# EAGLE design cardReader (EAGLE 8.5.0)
DELETE: MF
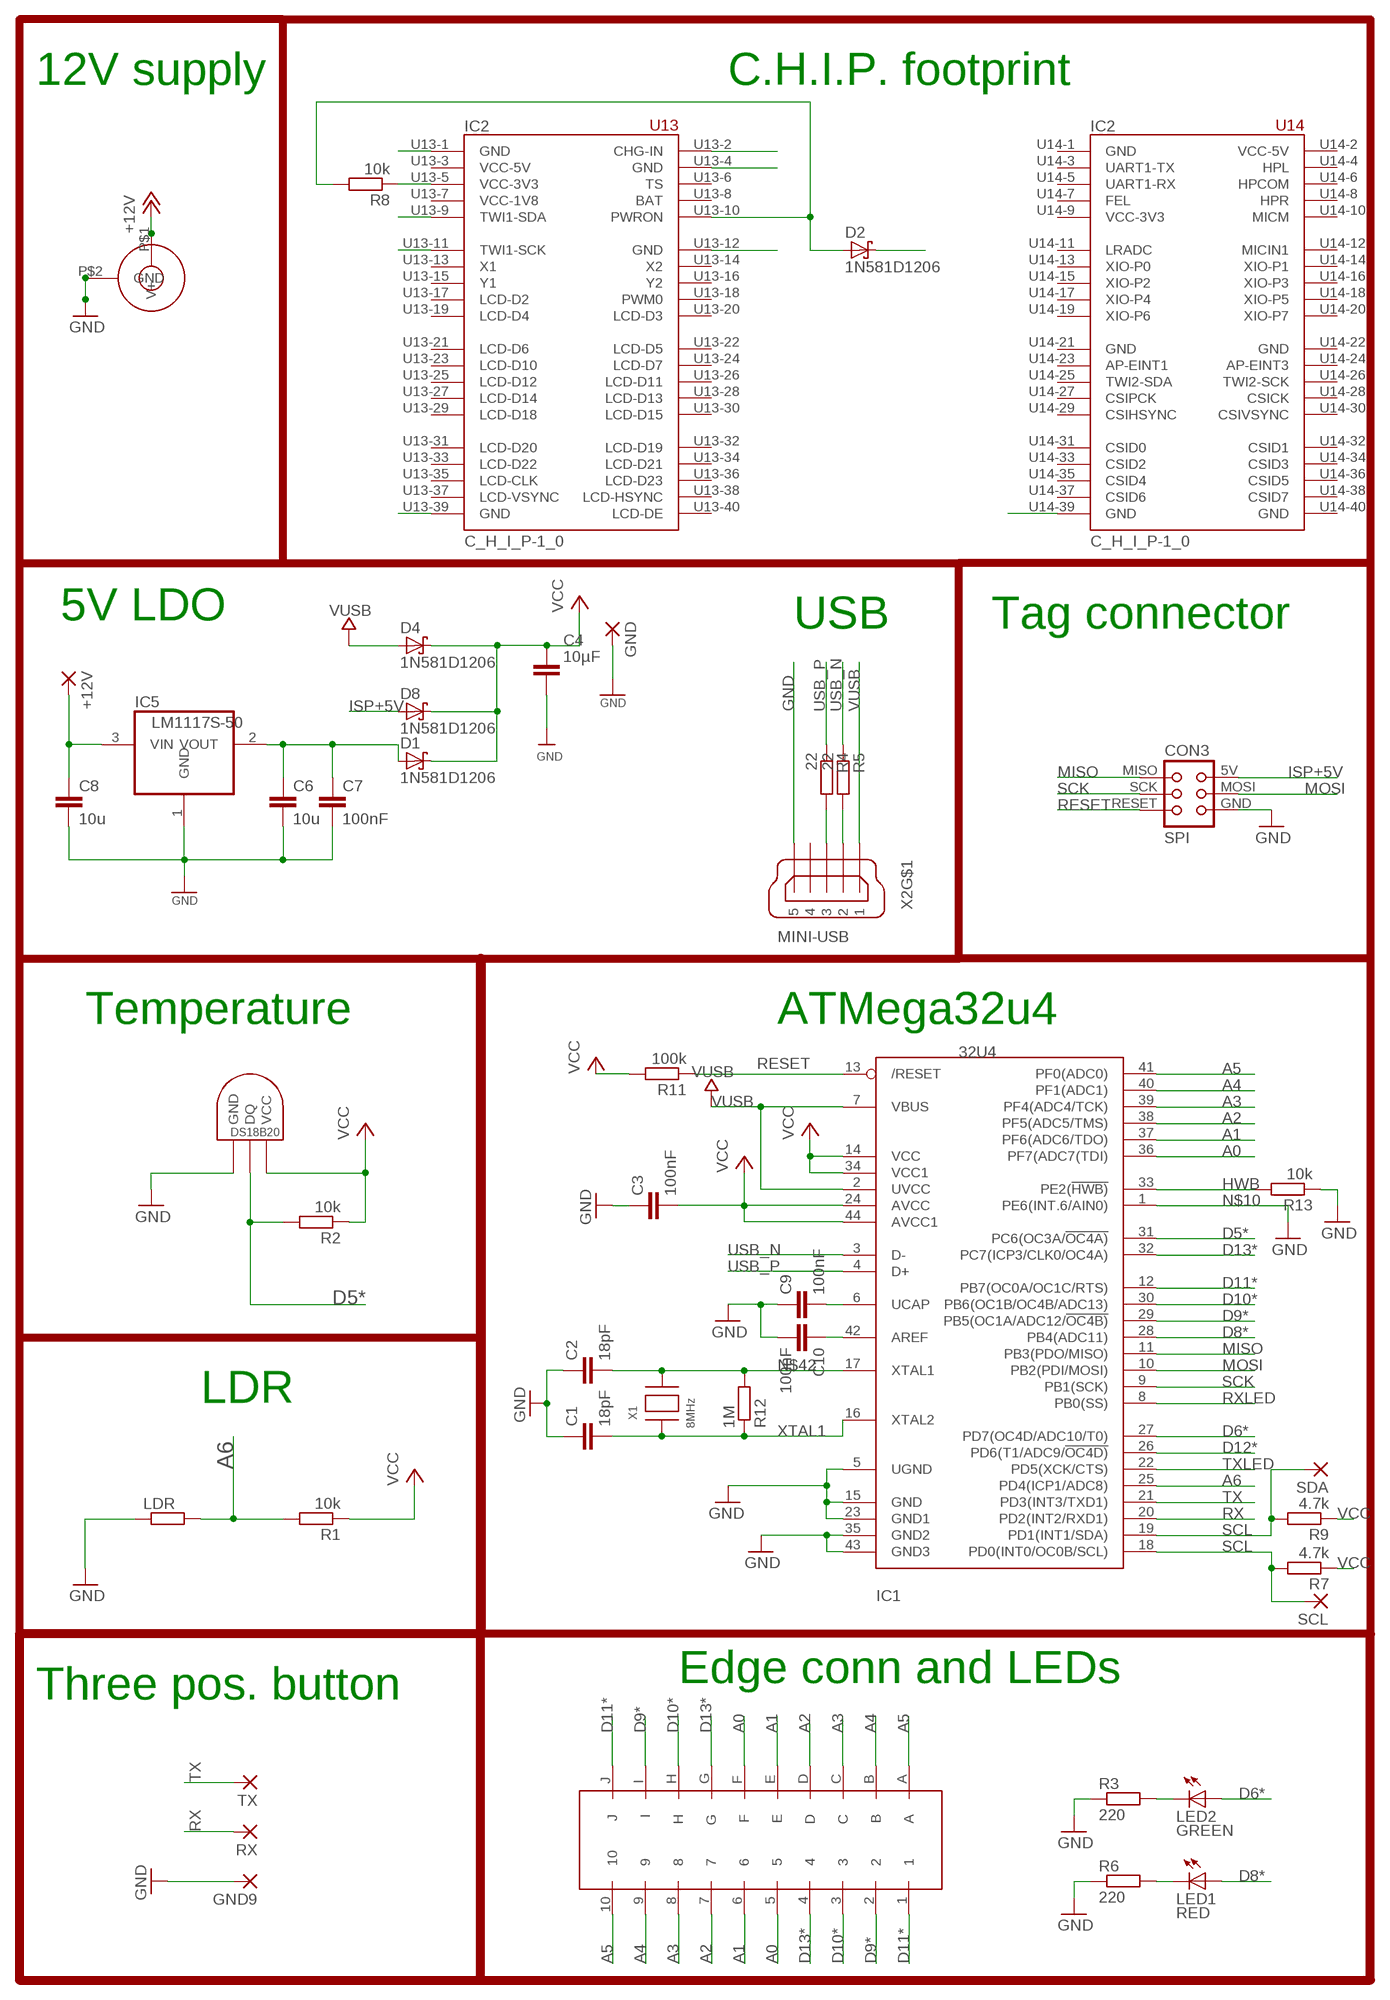
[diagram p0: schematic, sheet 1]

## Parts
+12V  SMD5  [SMD2,54-5,08]
C1  18pF  C-EUC0805K  [C0805K]
C2  18pF  C-EUC0805K  [C0805K]
C3  100nF  C-EUC0805K  [C0805K]
C4  10µF  CAPACITOR_NPOL-1206  [C1206]
C6  10u  C-EUC0805K  [C0805K]
C7  100nF  C-EUC0805K  [C0805K]
C8  10u  C-EUC0805K  [C0805K]
C9  100nF  C-EUC0805K  [C0805K]
C10  100nF  C-EUC0805K  [C0805K]
CON2  JACK_DC_BARREL  [DC_BARREL]
CON3  SPI  TINYISPT  [TC2030-MCP-NL]
D1  1N581D1206  [LED-1206]
D2  1N581D1206  [LED-1206]
D4  1N581D1206  [LED-1206]
D8  1N581D1206  [LED-1206]
GND  SMD5  [SMD2,54-5,08]
GND9  SMD5  [SMD2,54-5,08]
IC1  32U4  ATMEGA32U4-AU  [TQFP44]
IC2  C_H_I_P-1_0  [C_H_I_P-1_0]
IC5  LM1117S-50  REG1117  [SOT223]
LDR  R-EU_0207/2V  [0207/2V]
LED1  RED  LED5MM  [LED5MM]
LED2  GREEN  LED5MM  [LED5MM]
R1  10k  R-EU_R0805  [R0805]
R2  10k  R-EU_R0805  [R0805]
R3  220  R-EU_0204/7  [0204/7]
R4  22  R-EU_R0805  [R0805]
R5  22  R-EU_R0805  [R0805]
R6  220  R-EU_0204/7  [0204/7]
R7  4.7k  R-EU_R0805  [R0805]
R8  10k  R-EU_R0805  [R0805]
R9  4.7k  R-EU_R0805  [R0805]
R11  100k  R-EU_R0805  [R0805]
R12  1M  R-EU_R0805  [R0805]
R13  10k  R-EU_R0805  [R0805]
RX  SMD5  [SMD2,54-5,08]
SCL  SMD5  [SMD2,54-5,08]
SDA  SMD5  [SMD2,54-5,08]
TX  SMD5  [SMD2,54-5,08]
U$1  DS1820TO92  [DS1820]
U$3  CONN2X10PRINT  [CONN2X10PRINT]
X1  8MHz  XTALNX6035  [NX6035]
X2  MINI-USB  MINI-USB-SCHIELD-32005-201  [32005-201]

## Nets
+12V: +12V.1(P) C8.1 CON2.P$1(V+) IC5.3(VIN)
A0: IC1.36(PF7(ADC7(TDI)) U$3.5 U$3.F
A1: IC1.37(PF6(ADC6/TDO)) U$3.6 U$3.E
A2: IC1.38(PF5(ADC5/TMS)) U$3.7 U$3.D
A3: IC1.39(PF4(ADC4/TCK)) U$3.8 U$3.C
A4: IC1.40(PF1(ADC1)) U$3.9 U$3.B
A5: IC1.41(PF0(ADC0)) U$3.10 U$3.A
A6: IC1.25(PD4(ICP1/ADC8)) LDR.2 R1.2
AREF: C10.1 IC1.42(AREF)
D5*: IC1.31(PC6(OC3A/!OC4A)) R2.2 U$1.DQ
D6*: IC1.27(PD7(OC4D/ADC10/T0)) LED2.A
D8*: IC1.28(PB4(ADC11)) LED1.A
D9*: IC1.29(PB5(OC1A/ADC12/!OC4B)) U$3.2 U$3.I
D10*: IC1.30(PB6(OC1B/OC4B/ADC13)) U$3.3 U$3.H
D11*: IC1.12(PB7(OC0A/OC1C/RTS)) U$3.1 U$3.J
D12*: IC1.26(PD6(T1/ADC9/!OC4D))
D13*: IC1.32(PC7(ICP3/CLK0/OC4A)) U$3.4 U$3.G
GND [power]: C1.1 C2.1 C3.1 C4.2 C6.2 C7.2 C8.2 C9.1 C10.2 CON2.P$2(GND) CON3.GND GND9.1(P) GND.1(P) IC1.5(UGND) IC1.15(GND) IC1.23(GND1) IC1.35(GND2) IC1.43(GND3) IC2.U13-12(GND) IC2.U13-39(GND) IC5.1(GND) LDR.1 R3.1 R6.1 R13.1 U$1.GND X2.5
HWB: IC1.33(PE2(!HWB)) R13.2
ISP+5V: CON3.5V(VCC) D8.A
MISO: CON3.MISO IC1.11(PB3(PDO/MISO))
MOSI: CON3.MOSI IC1.10(PB2(PDI/MOSI))
N$1: C9.2 IC1.6(UCAP)
N$2: IC2.U13-2(CHG-IN)
N$3: LED2.K(C) R3.2
N$4: LED1.K(C) R6.2
N$5: IC2.U13-4(GND)
N$6: IC2.U13-1(GND)
N$7: IC2.U13-9(TWI1-SDA)
N$8: IC2.U13-11(TWI1-SCK)
N$9: C6.1 C7.1 D1.A IC5.2(VOUT)
N$10: D2.C IC1.1(PE6(INT.6/AIN0)) ; supply symbol labelled GND
N$11: IC2.U14-39(GND)
N$42: C2.2 IC1.17(XTAL1) R12.2 X1.P$2
PWRON: D2.A IC2.U13-10(PWRON) R8.2
RESET: CON3.RESET IC1.13(/RESET) R11.1
RX: IC1.20(PD2(INT2/RXD1)) RX.1(P)
RXLED: IC1.8(PB0(SS))
SCK: CON3.SCK IC1.9(PB1(SCK))
SCL: IC1.18(PD0(INT0/OC0B/SCL)) R7.2 SCL.1(P)
SDA: IC1.19(PD1(INT1/SDA)) R9.2 SDA.1(P)
TX: IC1.21(PD3(INT3/TXD1)) TX.1(P)
TXLED: IC1.22(PD5(XCK/CTS))
USB_N: IC1.3(D-) R5.1
USB_P: IC1.4(D+) R4.1
USBC_N: R5.2 X2.2
USBC_P: R4.2 X2.3
VCC: C3.2 C4.1 D1.C D4.C D8.C IC1.14(VCC) IC1.24(AVCC) IC1.34(VCC1) IC1.44(AVCC1) R1.1 R2.1 R7.1 R9.1 R11.2 U$1.VDD(VCC)
VCC-3V3@1: IC2.U13-5(VCC-3V3) R8.1
VUSB: D4.A IC1.2(UVCC) IC1.7(VBUS) X2.1
XTAL1: C1.2 IC1.16(XTAL2) R12.1 X1.P$1
Unconnected: IC2.U13-3(VCC-5V) IC2.U13-6(TS) IC2.U13-7(VCC-1V8) IC2.U13-13(X1) IC2.U13-14(X2) IC2.U13-15(Y1) IC2.U13-16(Y2) IC2.U13-17(LCD-D2) IC2.U13-18(PWM0) IC2.U13-19(LCD-D4) IC2.U13-20(LCD-D3) IC2.U13-21(LCD-D6) IC2.U13-22(LCD-D5) IC2.U13-23(LCD-D10) IC2.U13-24(LCD-D7) IC2.U13-25(LCD-D12) IC2.U13-26(LCD-D11) IC2.U13-27(LCD-D14) IC2.U13-28(LCD-D13) IC2.U13-29(LCD-D18) IC2.U13-30(LCD-D15) IC2.U13-31(LCD-D20) IC2.U13-32(LCD-D19) IC2.U13-33(LCD-D22) IC2.U13-34(LCD-D21) IC2.U13-35(LCD-CLK) IC2.U13-36(LCD-D23) IC2.U13-37(LCD-VSYNC) IC2.U13-38(LCD-HSYNC) IC2.U13-40(LCD-DE) IC2.U14-2(VCC-5V) IC2.U14-3(UART1-TX) IC2.U14-4(HPL) IC2.U14-5(UART1-RX) IC2.U14-6(HPCOM) IC2.U14-7(FEL) IC2.U14-8(HPR) IC2.U14-9(VCC-3V3) IC2.U14-10(MICM) IC2.U14-11(LRADC) IC2.U14-12(MICIN1) IC2.U14-13(XIO-P0) IC2.U14-14(XIO-P1) IC2.U14-15(XIO-P2) IC2.U14-16(XIO-P3) IC2.U14-17(XIO-P4) IC2.U14-18(XIO-P5) IC2.U14-19(XIO-P6) IC2.U14-20(XIO-P7) IC2.U14-23(AP-EINT1) IC2.U14-24(AP-EINT3) IC2.U14-25(TWI2-SDA) IC2.U14-26(TWI2-SCK) IC2.U14-27(CSIPCK) IC2.U14-28(CSICK) IC2.U14-29(CSIHSYNC) IC2.U14-30(CSIVSYNC) IC2.U14-31(CSID0) IC2.U14-32(CSID1) IC2.U14-33(CSID2) IC2.U14-34(CSID3) IC2.U14-35(CSID4) IC2.U14-36(CSID5) IC2.U14-37(CSID6) IC2.U14-38(CSID7) X2.4 X2.M1(S:S1) X2.M2(S:S2) X2.M3(S:S3) X2.M4(S:S4)

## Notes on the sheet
- 12V supply | C.H.I.P. footprint
- 5V LDO | USB | Tag connector
- Temperature | ATMega32u4
- LDR
- Edge conn and LEDs
- Three pos. button

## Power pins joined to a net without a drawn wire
BAT: IC2.U13-8(BAT)
GND: IC2.U14-1(GND) IC2.U14-21(GND) IC2.U14-22(GND) IC2.U14-40(GND)

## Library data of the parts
+12V GND GND9 RX SCL SDA TX = wirepad:SMD5: SMD PAD
C1 C2 = rcl:C-EU: CAPACITOR, European symbol; ELECROW: C1797; LCSC: C1797; MPN: 77-VJ1206A180JXXPBC
C3 C7 C9 C10 = rcl:C-EU: CAPACITOR, European symbol; ELECROW: C49678; LCSC: C49678; MPN: 80-C1206C104K5R
C4 = dp_devices:CAPACITOR_NPOL: Non-Polarized capacitor in various packages
C6 C8 = rcl:C-EU: CAPACITOR, European symbol; ELECROW: C15850; LCSC: C15850; MPN: 77-VJ1206V106ZXQTBC
CON2 = lpatiny:JACK_DC_BARREL
CON3 = lpatiny:TINYISP: CONNECTOR
D1 D2 D4 D8 = lpatiny:1N581*: 1.0A SCHOTTKY BARRIER RECTIFIER
IC1 = adafruit:ATMEGA32U4: http://www.ladyada.net/library/eagle; LCSC: C44854; MPN: 556-ATMEGA32U4RC-AU
IC2 = SENG:C_H_I_P-1_0: C.H.I.P. 1.0 Linux computer module with on chip power management unit
IC5 = burr-brown:REG1117: 800mA and 1A Low Dropout (LDO) Positive Regulator 1.8V, 2.5V, 2.85V, 3.3V, 5V, and Adj; LCSC: C126027; MPN: REG1117; OC_FARNELL: 1097566; OC_NEWARK: 14P6981
LDR R3 R6 = rcl:R-EU_: RESISTOR, European symbol
LED1 LED2 = SparkFun:LED: LEDs
R1 R2 R7-R9 R11 = rcl:R-EU_: RESISTOR, European symbol; ELECROW: C17407; LCSC: C17407; MPN: RC1206FR-07100KL
R4 R5 = rcl:R-EU_: RESISTOR, European symbol; ELECROW: C17561; LCSC: C17561
R12 = rcl:R-EU_: RESISTOR, European symbol; ELECROW: C17514; LCSC: C17514
R13 = rcl:R-EU_: RESISTOR, European symbol; ELECROW: C17414; LCSC: C17414
U$1 = Ava:DS1820: DS18B20 Programmable Resolution 1-Wire Digital Thermometer Description The DS18B20 digital thermometer provides 9-bit to 12-bit Celsius temperature measurements and has an alarm function with nonvolatile user-programmable upper and lower trigger points. The DS18B20 communicates over a 1-Wire® bus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
U$3 = edgeConn2x10:CONN2X10PRINT: Footprint for 10/20 edge connector.
X1 = lpatiny:XTAL: Low cost SMT crystals, no capacitors included; LCSC: C122522; MPN: 729-F60800010
X2 = con-cypressindustries:MINI-USB-SCHIELD-: MINI USB-B Conector Source: www.cypressindustries.com; LCSC: C46391; MPN: 649-10033526-N3212LF

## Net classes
0 default: width 0.254 mm, clearance 0.25 mm
1 power: width 0.254 mm, drill 0.305 mm, clearance 0.25 mm
2 VIN: width 0.254 mm, clearance 0.25 mm
3 fine: width 0.254 mm, clearance 0.25 mm
4 aref: width 0.254 mm, clearance 0.25 mm

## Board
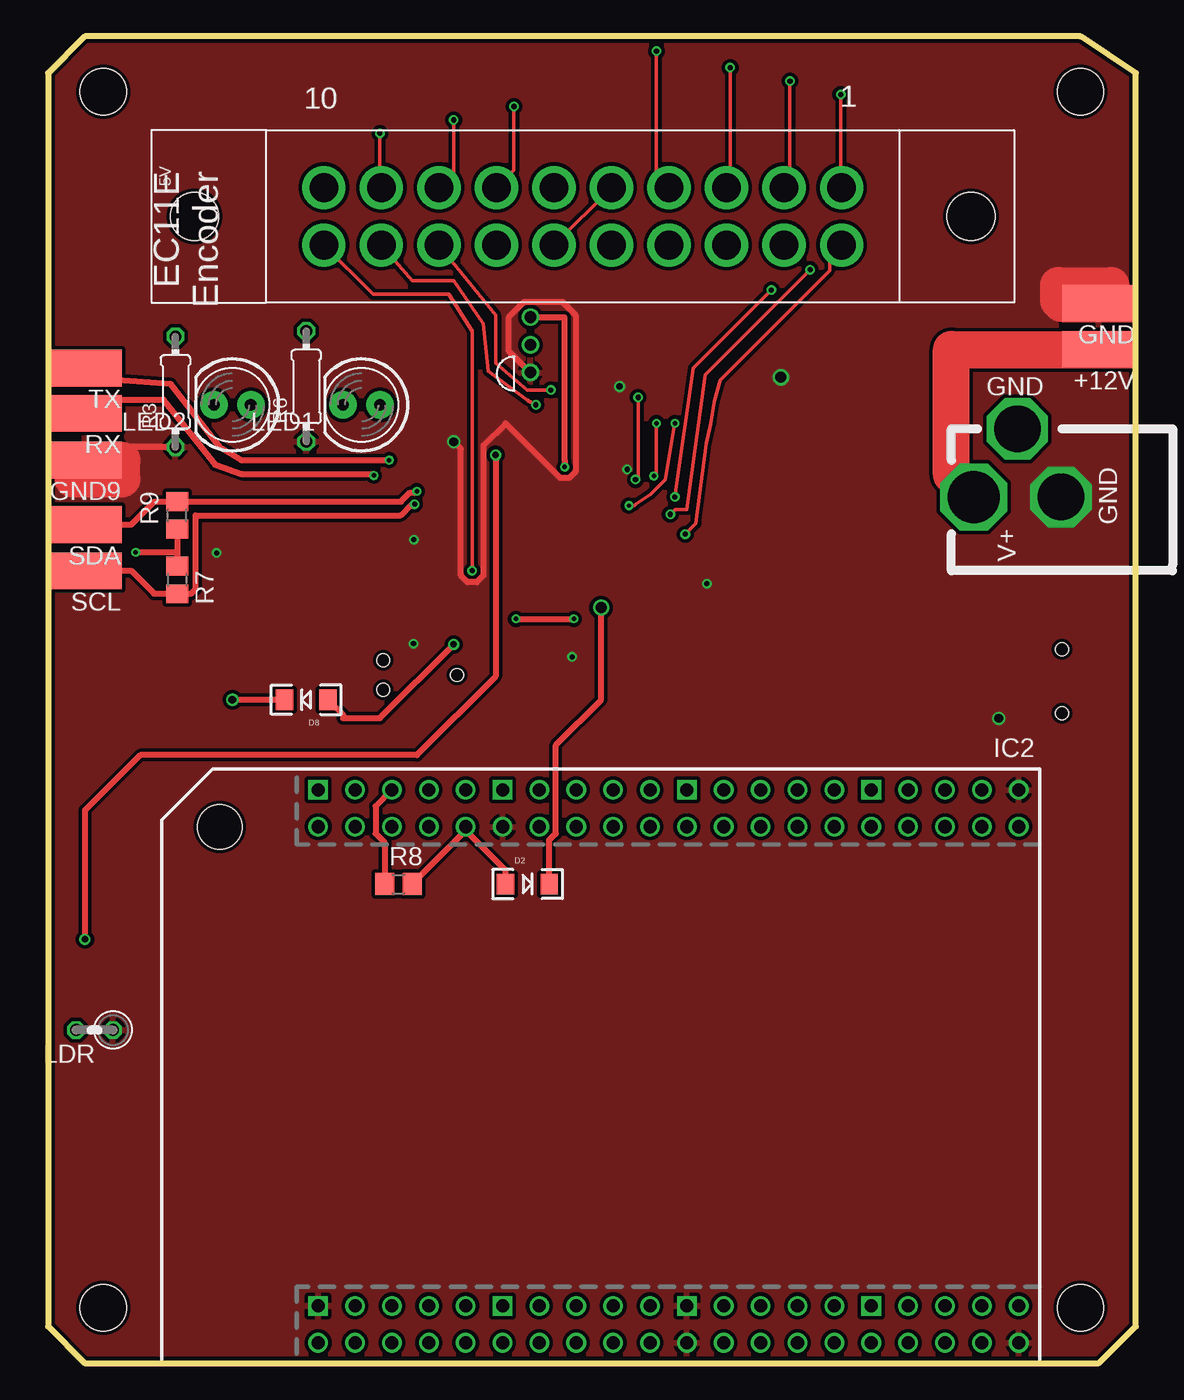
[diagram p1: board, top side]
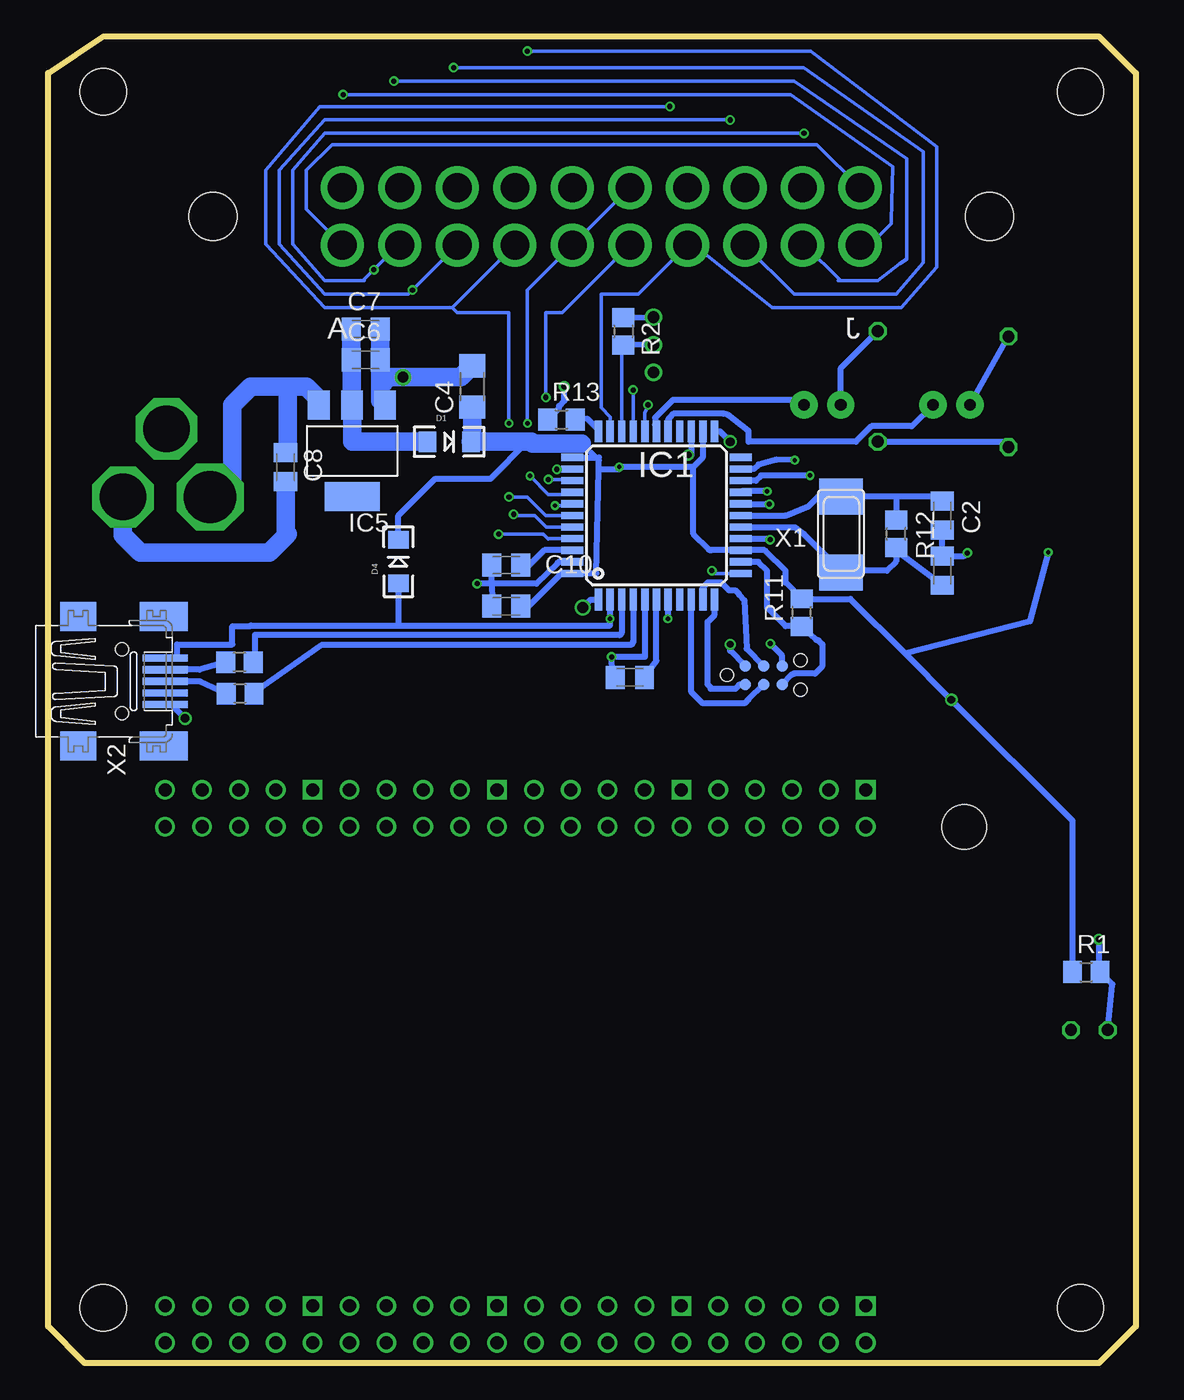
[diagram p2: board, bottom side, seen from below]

Size 74.93 x 91.44 mm. Coordinates in mm from the lower left corner, seen from the top.
Outline: 0,88.9 0,2.54 2.54,0 72.39,0 74.93,2.54 74.93,88.9 71.12,91.44 2.54,91.44 0,88.9
Copper layers (1*2*15*16): Top 0.035mm / dielectric 0.2mm / layer 2 0.0175mm / dielectric 1.1mm / layer 15 0.0175mm / dielectric 0.2mm / Bottom 0.035mm
Design rules "SeeedStudio_DRU_no_angle_20130527": minimum track width 6mil, minimum drill 12mil, track to track 6mil, track to pad 6mil, pad to pad 6mil, via to via 6mil, smd to smd 0mil, copper to edge 10mil, drill to drill 10mil, minimum pad ring 6mil, minimum via ring 6mil, stop-mask expansion 2mil, vias tented up to drill 25mil, thermal gap 10mil
Holes 3.2 mm at 3.81,87.63 3.81,3.81 71.12,87.63 71.12,3.81

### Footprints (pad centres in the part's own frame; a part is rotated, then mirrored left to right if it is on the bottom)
SMD2,54-5,08 = smd 2.54 x 5.08: 1 0,0
C0805K = smd 1.3 x 1.6: 1 -1,0; 2 1,0
C1206 = smd 1.6 x 1.803: 1 -1.422,0; 2 1.422,0
DC_BARREL = drill 3.6 pad 4.5 octagon: P$1 0,13.7 | drill 3.2 pad 4.064 octagon: P$2 0,7.7; P$3 4.7,10.7
TC2030-MCP-NL = smd 0.787 x 0.787: 5V 1.27,0.635; GND 3.81,0.635; MISO 1.27,-0.635; MOSI 2.54,0.635; RESET 3.81,-0.635; SCK 2.54,-0.635 | hole 0.889: 0,0; 5.08,-1.016; 5.08,1.016
LED-1206 = smd 1.2 x 1.4: A -1.5,0; C 1.5,0
TQFP44 = smd 1.5 x 0.5: 1 -5.8,4; 2 -5.8,3.2; 3 -5.8,2.4; 4 -5.8,1.6; 5 -5.8,0.8; 6 -5.8,0; 7 -5.8,-0.8; 8 -5.8,-1.6; 9 -5.8,-2.4; 10 -5.8,-3.2; 11 -5.8,-4; 23 5.8,-4; 24 5.8,-3.2; 25 5.8,-2.4; 26 5.8,-1.6; 27 5.8,-0.8; 28 5.8,0; 29 5.8,0.8; 30 5.8,1.6; 31 5.8,2.4; 32 5.8,3.2; 33 5.8,4 | smd 0.5 x 1.5: 12 -4,-5.8; 13 -3.2,-5.8; 14 -2.4,-5.8; 15 -1.6,-5.8; 16 -0.8,-5.8; 17 0,-5.8; 18 0.8,-5.8; 19 1.6,-5.8; 20 2.4,-5.8; 21 3.2,-5.8; 22 4,-5.8; 34 4,5.8; 35 3.2,5.8; 36 2.4,5.8; 37 1.6,5.8; 38 0.8,5.8; 39 0,5.8; 40 -0.8,5.8; 41 -1.6,5.8; 42 -2.4,5.8; 43 -3.2,5.8; 44 -4,5.8
C_H_I_P-1_0 = drill 0.9 square: U13-1 0,0; U13-11 -12.7,0; U13-21 -25.4,0; U13-31 -38.1,0; U14-1 0,35.56; U14-11 -12.7,35.56; U14-21 -25.4,35.56; U14-31 -38.1,35.56 | drill 0.9: U13-2 0,2.54; U13-3 -2.54,0; U13-4 -2.54,2.54; U13-5 -5.08,0; U13-6 -5.08,2.54; U13-7 -7.62,0; U13-8 -7.62,2.54; U13-9 -10.16,0; U13-10 -10.16,2.54; U13-12 -12.7,2.54; U13-13 -15.24,0; U13-14 -15.24,2.54; U13-15 -17.78,0; U13-16 -17.78,2.54; U13-17 -20.32,0; U13-18 -20.32,2.54; U13-19 -22.86,0; U13-20 -22.86,2.54; U13-22 -25.4,2.54; U13-23 -27.94,0; U13-24 -27.94,2.54; U13-25 -30.48,0; U13-26 -30.48,2.54; U13-27 -33.02,0; U13-28 -33.02,2.54; U13-29 -35.56,0; U13-30 -35.56,2.54; U13-32 -38.1,2.54; U13-33 -40.64,0; U13-34 -40.64,2.54; U13-35 -43.18,0; U13-36 -43.18,2.54; U13-37 -45.72,0; U13-38 -45.72,2.54; U13-39 -48.26,0; U13-40 -48.26,2.54; U14-2 0,38.1; U14-3 -2.54,35.56; U14-4 -2.54,38.1; U14-5 -5.08,35.56; U14-6 -5.08,38.1; U14-7 -7.62,35.56; U14-8 -7.62,38.1; U14-9 -10.16,35.56; U14-10 -10.16,38.1; U14-12 -12.7,38.1; U14-13 -15.24,35.56; U14-14 -15.24,38.1; U14-15 -17.78,35.56; U14-16 -17.78,38.1; U14-17 -20.32,35.56; U14-18 -20.32,38.1; U14-19 -22.86,35.56; U14-20 -22.86,38.1; U14-22 -25.4,38.1; U14-23 -27.94,35.56; U14-24 -27.94,38.1; U14-25 -30.48,35.56; U14-26 -30.48,38.1; U14-27 -33.02,35.56; U14-28 -33.02,38.1; U14-29 -35.56,35.56; U14-30 -35.56,38.1; U14-32 -38.1,38.1; U14-33 -40.64,35.56; U14-34 -40.64,38.1; U14-35 -43.18,35.56; U14-36 -43.18,38.1; U14-37 -45.72,35.56; U14-38 -45.72,38.1; U14-39 -48.26,35.56; U14-40 -48.26,38.1 | hole 3.08: 6.78,2.56
SOT223 = smd 1.499 x 2.007: 1 -2.261,-3.15; 2 0.025,-3.15; 3 2.311,-3.15 | smd 3.81 x 2.007: 4 0,3.15
0207/2V = drill 0.813 octagon: 1 -1.27,0; 2 1.27,0
LED5MM = drill 0.813 pad 1.88: A -1.27,0; K 1.27,0
R0805 = smd 1.3 x 1.5: 1 -0.95,0; 2 0.95,0
0204/7 = drill 0.813 octagon: 1 -3.81,0; 2 3.81,0
DS1820 = drill 0.8: DQ 2.54,-1.27; GND 0.635,-1.27; VDD 4.445,-1.27
CONN2X10PRINT = drill 1.981: 1 17.831,1.981; 2 13.868,1.981; 3 9.906,1.981; 4 5.944,1.981; 5 1.981,1.981; 6 -1.981,1.981; 7 -5.944,1.981; 8 -9.906,1.981; 9 -13.868,1.981; 10 -17.831,1.981; A 17.831,-1.981; B 13.868,-1.981; C 9.906,-1.981; D 5.944,-1.981; E 1.981,-1.981; F -1.981,-1.981; G -5.944,-1.981; H -9.906,-1.981; I -13.868,-1.981; J -17.831,-1.981 | hole 3.302: -26.746,0; 26.746,0
NX6035 = smd 2.5 x 3: P$1 2.665,0; P$2 -2.565,0
32005-201 = smd 3.1 x 0.5: 1 3,1.6; 2 3,0.8; 3 3,0; 4 3,-0.8; 5 3,-1.6 | smd 2.5 x 2: M1 -3,-4.45; M2 -3,4.45 | smd 3.3 x 2: M3 2.9,4.45; M4 2.9,-4.45 | hole 0.9: 0,2.2; 0,-2.2

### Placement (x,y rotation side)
+12V  72.39,69.85 90 top
C1  13.34,54.61 270 bottom
C2  13.34,58.42 90 bottom
C3  43.37,52.17 0 bottom
C4  45.72,67.31 90 bottom
C6  53.05,69.14 0 bottom
C7  53.05,71.26 0 bottom
C8  58.57,61.76 270 bottom
C9  34.85,47.26 0 bottom
C10  43.37,55 180 bottom
CON2  77.47,59.69 90 top
CON3  28.17,47.42 0 bottom
D1  47.31,63.5 0 bottom
D2  33.02,33.02 0 top
D4  50.8,55.24 90 bottom
D8  17.78,45.72 180 top
GND  72.39,73.02 90 top
GND9  2.54,62.23 90 top
IC1  33.02,58.42 90 bottom
IC2  18.61,39.51 180 top
IC5  53.98,62.87 180 bottom
LDR  3.2,22.96 180 top
LED1  21.59,66.04 180 top
LED2  12.7,66.04 180 top
R1  3.42,26.96 0 bottom
R2  35.31,71.11 270 bottom
R3  8.78,66.94 90 top
R4  61.7,46.14 180 bottom
R5  61.75,48.31 180 bottom
R6  17.78,67.31 90 top
R7  8.89,53.98 270 top
R8  24.13,33.02 0 top
R9  8.89,58.42 90 top
R11  23.01,51.73 90 bottom
R12  16.51,57.15 90 bottom
R13  39.57,65.02 0 bottom
RX  2.54,65.46 90 top
SCL  2.54,54.61 90 top
SDA  2.54,57.79 90 top
TX  2.54,68.58 90 top
U$1  31.95,67.64 90 top
U$3  36.83,79.03 0 top
X1  20.32,57.15 270 bottom
X2  69.85,46.99 0 bottom

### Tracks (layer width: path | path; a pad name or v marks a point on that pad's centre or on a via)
+12V
  Top 1.27: 71.12,69.85 +12V.1
  Top 2.54: CON2.P$1 62.23,61.23 62.23,69.85 71.12,69.85
  Bottom 1.27: IC5.3 56.29,66.34 arc-45 56.36,66.52 57.15,67.31 58.42,67.31 | 58.42,67.31 60.96,67.31 62.23,66.04 62.23,60.96 62.5,60.96 CON2.P$1 | C8.1 58.42,62.91 58.42,67.31
A0  (via drill 0.35)
  Top 0.254: U$3.F U$3.5 | v40.64,66.56 40.64,60.96 40.58,60.9 v40.46,60.9
  Bottom 0.254: U$3.F 39.51,72.39 40.64,72.39 v40.64,66.56 | v40.46,60.9 38.9,60.9 IC1.36
A1  (via drill 0.3)
  Top 0.254: v41.91,64.77 41.91,61.32 v41.73,61.14
  Bottom 0.254: U$3.6 U$3.E 41.91,73.95 v41.91,64.77 | 39.78,59.87 39.39,59.93 | 39.39,59.93 IC1.37 | v41.73,61.14 40.46,59.87 39.45,59.87 39.39,59.93
A2  (via drill 0.3, 0.35)
  Top 0.254: v32.09,86.6 32.09,82.22 U$3.7 | v43.18,64.77 42.53,60.91 41.49,59.87 40.46,59.18 40.38,59.1 v40.01,59.1
  Bottom 0.254: 47.09,72.73 55.88,72.73 59.93,77.13 59.93,82.21 56.22,86.6 v32.09,86.6 | U$3.D 47.09,72.73 | 47.09,72.73 46.75,72.39 43.18,72.39 v43.18,64.77 | v40.01,59.1 38.94,59.1 IC1.38
A3  (via drill 0.35)
  Top 0.254: v27.94,85.67 27.94,82.03 U$3.8 | v49.83,73.96 44.45,68.58 v43.18,59.69
  Bottom 0.254: v27.94,85.67 55.88,85.67 59,82.21 59,77.13 55.88,73.66 50.13,73.66 v49.83,73.96 U$3.C | v43.18,59.69 41.91,59.69 40.64,58.42 IC1.39
A4  (via drill 0.35)
  Top 0.254: v22.86,84.75 22.86,81.11 U$3.9 | v42.86,58.5 43.2,58.84 43.99,58.84 45.26,68.12 v52.49,75.35
  Bottom 0.254: 53.16,74.59 53.25,74.59 | 53.25,74.59 55.88,74.59 58.08,77.13 58.08,82.21 55.88,84.75 v22.86,84.75 | 53.25,74.59 v52.49,75.35 50.79,77.05 U$3.B | v42.86,58.5 42.79,58.42 41.41,58.42 40.62,57.62 IC1.40
  Bottom 0.406: 38.82,57.66 IC1.40
A5  (via drill 0.35)
  Top 0.254: U$3.A 53.84,76.22 53.84,75.3 46.29,67.75 45.9,66.27 45.65,64.75 45.34,63.36 44.62,57.88 44.62,57.85 v43.89,57.12
  Bottom 0.254: U$3.10 21.97,83.98 55.37,83.98 57.15,82.21 57.15,79.54 U$3.A | v43.89,57.12 40.83,57.12 40.82,57.12 40.8,57.12 40.46,56.78 40.42,56.82 IC1.41
A6  (via drill 0.45)
  Top 0.406: v30.82,62.59 30.82,47.33 25.4,41.91 6.35,41.91 2.54,38.1 v2.54,29.21
  Bottom 0.406: LDR.2 1.61,26.11 R1.2 2.54,27.04 v2.54,29.21 | IC1.25 30.62,62.55 30.71,62.46 30.71,62.48 v30.82,62.59
AREF
  Bottom 0.406: C10.1 42.19,54.82 arc-45 42.01,54.75 40.74,56.02 IC1.42
D5*
  Bottom 0.254: R2.2 35.42,70.04 IC1.31
  Bottom 0.406: 35.43,64.22 IC1.31 | U$1.DQ R2.2
D6*
  Bottom 0.406: LED2.A 15.45,64.56 18.22,64.56 19.28,63.5 26.67,63.5 26.67,64.25 28.12,65.35 28.39,65.42 31.86,65.42 32.12,65.16 32.12,65.12 32.23,65.01 32.22,65 IC1.27
D8*
  Bottom 0.406: LED1.A 23.2,66.38 31.89,66.38 33.12,65.16 33.12,64.67 33.02,64.57 IC1.28
D9*  (via drill 0.35)
  Top 0.254: v51.1,88.35 51.1,81.42 U$3.2 | U$3.I 25.08,74.59 27.94,74.59 29.98,71.62 30.32,68.37 32.99,66.38 v33.6,66.04
  Bottom 0.254: 20.5,74.59 20.33,74.59 | 20.33,74.59 17.78,74.59 16.27,75.76 15.79,76.1 15.79,82.99 23.55,88.35 v51.1,88.35 | 20.33,74.59 22.8,77.05 U$3.I | v33.6,66.04 33.82,65.48 IC1.29
D10*  (via drill 0.35)
  Top 0.254: v46.99,89.28 46.99,81.27 U$3.3 | U$3.H 30.82,72.22 30.82,68.92 33.02,67.07 v34.63,67.07
  Bottom 0.254: v46.99,89.28 22.86,89.28 14.66,83.48 14.66,75.86 16.51,73.66 23.53,73.66 U$3.H | v34.63,67.07 34.62,65.71 IC1.30
D11*  (via drill 0.35)
  Top 0.254: v54.61,87.43 54.61,81.06 U$3.1 | U$3.J 22.39,73.66 27.6,73.66 29.21,71.12 v29.21,54.61
  Bottom 0.254: v54.61,87.43 23.79,87.43 16.75,82.45 16.85,78.75 16.85,78.51 18.31,77.05 U$3.J | v29.21,54.61 29.02,54.42 IC1.12
D13*  (via drill 0.35)
  Top 0.254: v41.91,90.41 41.91,81.88 U$3.4
  Bottom 0.254: v41.91,90.41 22.38,90.41 13.73,83.82 13.73,75.51 16.17,72.73 25.06,72.73 30.4,77.05 U$3.G 34.28,73.66 36.83,73.66 36.83,65.84 36.2,65.2 36.2,64.22
  Bottom 0.406: 36.2,64.22 IC1.32
GND  (via drill 0.35, 0.45, 0.6, 0.75)
  Top 0.406: R3.1 3.44,63.13 GND9.1 | U$1.GND 31.75,69.75 31.75,72.1 32.79,73.14 35.44,73.14 36.34,72.23 36.34,61.45 35.9,61 35.27,61 31.51,64.76 29.99,63.24 29.99,54.29 29.53,53.83 28.89,53.83 28.43,54.29 28.43,63.01 v27.94,63.5
  Top 2.54: GND9.1 1.73,61.42 1.73,60.96 5.08,60.96 5.08,62.23 | GND.1 69.83,73.02 69.61,73.24 69.61,74.27 73.2,74.27
  Bottom 0.254: IC1.35 38.86,61.58 39.78,61.58 39.8,61.6 v39.89,61.6
  Bottom 0.406: IC1.15 25.47,56.82 arc45 25.29,56.75 25.25,56.7 v25.2,56.76 | v11.61,55.84 11.77,55.68 arc45 11.95,55.61 C1.1 C2.1 | IC1.5 33.82,50.88 | 33.82,50.88 arc45 33.82,50.88 | IC1.43 39.66,55.22 arc-45 39.84,55.15 41.29,53.72 44.37,53.72 | 44.37,53.72 44.35,54.95 arc-45 C10.2 | 44.37,53.72 44.35,52.57 arc45 C3.1 | 44.37,53.72 v45.38,53.72 | CON3.GND 24.36,48.77 v25.17,49.58 | C9.1 36.07,47.6 v36.11,48.67 33.82,48.67 33.82,50.88 | X2.5 66.45,45.39 v65.49,44.44 | R6.1 9.14,63.5 R3.1 | IC1.23 28.66,64.22 v27.94,63.5 | R13.1 39.73,65.82 39.73,65.96 39.37,66.32 v39.37,67.31
  Bottom 1.27: CON2.P$2 69.77,57.07 68.58,55.88 59.69,55.88 58.42,57.15 58.57,57.3 C8.2 | C7.2 C6.2 52.05,67.31 | 52.05,67.31 52.05,66.35 IC5.1 | 52.05,67.31 51.41,67.94 v50.48,67.94 46.51,67.94 C4.2
  pour Top: 0,88.9 0,2.54 2.54,0 72.39,0 74.93,2.54 74.93,88.9 71.12,91.44 2.54,91.44
HWB
  Bottom 0.406: IC1.33 37.02,64.32 37.78,65.09 R13.2
ISP+5V  (via drill 0.45)
  Top 0.406: v27.94,49.53 22.86,44.45 20.32,44.45 20.32,44.68 D8.A
  Bottom 0.406: CON3.5V 27.94,49.1 v27.94,49.53
MISO
  Bottom 0.406: CON3.MISO 27.17,46.79 arc-45 27.35,46.71 27.57,46.49 29.21,46.49 | 29.29,46.49 29.21,46.49 | IC1.11 arc-45 IC1.11 29.02,51.56 29.49,51.09 29.49,46.77 29.21,46.49
MOSI
  Bottom 0.406: IC1.10 29.82,53.46 29.46,53.82 28.58,53.82 28.03,53.27 27.6,53.27 27.33,53.01 27.33,52.96 26.96,52.59 26.81,49.24 CON3.MOSI
N$1
  Bottom 0.406: C9.2 33.02,48.39 IC1.6
N$3
  Bottom 0.406: LED2.K R3.2
N$4
  Bottom 0.406: LED1.K 20.32,68.58 R6.2
N$9
  Bottom 1.27: D1.A 53.98,63.5 53.98,65.99 IC5.2 54,69.09 C6.1 C7.1
N$10  (via drill 0.75)
  Top 0.406: D2.C 34.52,36.05 34.97,36.5 34.97,42.59 38.1,45.72 v38.1,52.07
  Bottom 0.406: v38.1,52.07 37.55,52.62 IC1.1
N$42
  Bottom 0.406: IC1.17 24.13,58.42 22.54,59.05 21.91,59.69 20.32,59.69 X1.P$2 16.51,59.72 | 16.51,59.72 R12.2 | C2.2 13.58,59.72 16.51,59.72
PWRON
  Top 0.406: R8.2 28.77,36.7 | 28.77,36.7 IC2.U13-10 | D2.A 31.52,33.95 28.77,36.7
RESET
  Bottom 0.406: CON3.RESET 23.7,47.45 arc45 23.52,47.52 22.09,47.52 21.66,47.94 arc-45 21.59,48.12 21.59,49.53 21.84,49.78 arc-45 22.02,49.85 R11.1 23.04,50.8 24.13,50.8 25.4,52.07 25.4,54.61 26.01,55.22 IC1.13
RX  (via drill 0.3)
  Top 0.406: RX.1 2.21,66.42 7.95,66.42 11.5,61.91 13.34,61.28 22.34,61.28 v22.44,61.18
  Bottom 0.406: IC1.20 26.18,60.82 25.82,61.18 v22.44,61.18
SCK
  Bottom 0.406: CON3.SCK 26.68,45.73 26.84,45.58 26.95,45.47 29.83,45.47 30.62,46.25 IC1.9
SCL  (via drill 0.35)
  Top 0.406: 25.25,59.11 25.18,59.04 arc45 v25.25,59.2 25.06,59.2 24.28,58.42 10.16,58.42 10.16,53.34 9.85,53.02 R7.2 7.3,53.02 5.71,54.61 SCL.1
  Bottom 0.406: IC1.18 25.47,59.22 arc45 25.29,59.15 25.25,59.11 v25.25,59.2
SDA  (via drill 0.3)
  Top 0.406: SDA.1 5.71,57.79 7.3,59.37 R9.2 24.3,59.37 24.91,59.98 25.4,59.98 v25.4,60.08
  Bottom 0.406: v25.4,60.08 27.16,60.08 IC1.19
TX  (via drill 0.3)
  Top 0.406: TX.1 4.26,67.81 8.43,67.5 11.79,63.18 13.34,62.23 v23.5,62.23
  Bottom 0.406: v23.5,62.23 24.74,62.25 25.99,61.94 26.3,61.62 IC1.21
USB_N
  Bottom 0.254: R5.1 60.74,48.31 60.69,48.26
  Bottom 0.406: IC1.3 35.42,50.3 35.56,50.16 35.59,50.19 60.69,50.19 60.69,48.26 60.69,48.21
USB_P
  Bottom 0.406: IC1.4 34.62,49.76 arc90 34.87,49.51 56.07,49.51 60.39,46.46 R4.1
USBC_N
  Bottom 0.406: R5.2 64.49,47.79 X2.2
USBC_P
  Bottom 0.406: R4.2 64.45,46.99 X2.3 67.31,46.99
VCC  (via drill 0.3, 0.55)
  Top 0.406: U$1.VDD 35.56,72.08 35.56,62.23 35.59,62.23 v35.59,61.76 | R9.1 8.89,55.88 | 8.89,55.88 R7.1 | 8.89,55.88 v6.03,55.88 | D8.C v12.7,45.72
  Bottom 0.406: 36.99,61.6 37.17,54.42 IC1.44 39.45,54.42 arc-45 39.63,54.35 41.91,52.07 arc45 41.94,52.08 C3.2 | 36.99,61.6 36.99,62.23 | 36.99,62.23 36.99,62.42 IC1.34 | IC1.24 29.84,64.22 29.84,62.4 30.48,61.76 | 30.48,61.76 v35.59,61.76 35.59,61.6 36.99,61.6 | 30.48,61.76 30.48,57.15 29.42,56.09 arc-45 29.25,56.02 IC1.14 25.57,56.02 25.52,55.98 25.5,55.98 24.13,54.61 24.13,53.8 R11.2 19.66,52.68 15.88,48.9 | R2.1 U$1.VDD | R1.1 4.37,37.39 v12.7,45.72 15.88,48.9 | 36.99,62.23 38.15,63.39 38.16,63.39 | v6.03,55.88 7.3,51.12 15.88,48.9 | D4.C 50.8,58.42 48.26,60.96 44.45,60.96 41.91,63.5 41.65,63.5
  Bottom 1.27: 38.16,63.39 41.54,63.39 41.65,63.5 D1.C 45.72,63.59 C4.1
VCC-3V3@1
  Top 0.406: R8.1 23.18,35.88 22.56,36.5 22.56,38.38 IC2.U13-5
VUSB  (via drill 0.3)
  Top 0.406: v32.23,51.3 v36.22,51.3
  Bottom 0.406: X2.1 66.04,48.59 66.04,49.53 62.23,49.53 62.23,50.8 61.01,50.8 60.97,50.85 50.8,50.85 | 50.8,50.85 36.22,50.85 v36.22,51.3 IC1.2 | v32.23,51.3 v32.22,51.3 IC1.7 | D4.A 50.8,50.85
XTAL1
  Bottom 0.406: 20.32,54.61 17.14,54.61 16.51,55.24 R12.1 16.51,56.01 C1.2 | 20.32,54.61 X1.P$1 | 20.32,54.61 22.86,57.15 23.5,57.62 IC1.16

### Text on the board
tNames: EC11E / Encoder | 5V
tValues: Card Reader - v1.0.0
bValues: Card Reader - v1.0.0

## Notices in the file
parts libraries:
lpatiny: ©2009 ROFA.cz - modified and updated by Robert Darlington ‹rdarlington@gmail.com›
SparkFun: Licensing: CC v3.0 Share-Alike You are welcome to use this library for commercial purposes.
